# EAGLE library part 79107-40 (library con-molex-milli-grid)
RECEPTACAL
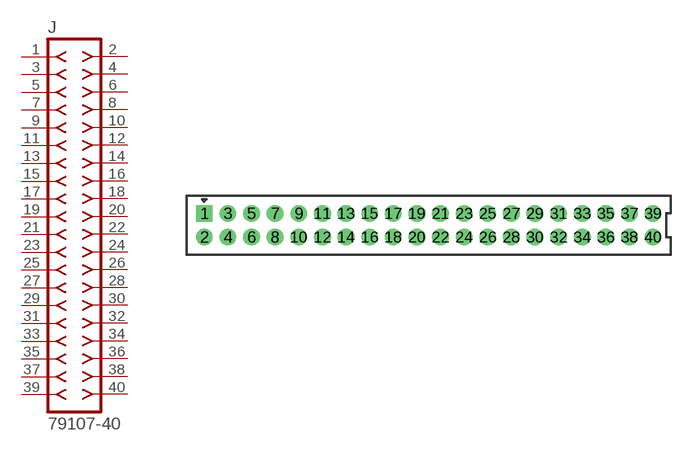
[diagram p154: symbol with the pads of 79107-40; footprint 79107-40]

Designator prefix J

## 79107-40  [79107-40]
1  1  pas
2  2  pas
3  3  pas
4  4  pas
5  5  pas
6  6  pas
7  7  pas
8  8  pas
9  9  pas
10  10  pas
11  11  pas
12  12  pas
13  13  pas
14  14  pas
15  15  pas
16  16  pas
17  17  pas
18  18  pas
19  19  pas
20  20  pas
21  21  pas
22  22  pas
23  23  pas
24  24  pas
25  25  pas
26  26  pas
27  27  pas
28  28  pas
29  29  pas
30  30  pas
31  31  pas
32  32  pas
33  33  pas
34  34  pas
35  35  pas
36  36  pas
37  37  pas
38  38  pas
39  39  pas
40  40  pas

## Footprint 79107-40 (pad centres in mm)
RECEPTACAL Dual Row, Vertical, Through-Hole
drill 0.914 square: 1 -19,1
drill 0.914: 2 -19,-1; 3 -17,1; 4 -17,-1; 5 -15,1; 6 -15,-1; 7 -13,1; 8 -13,-1; 9 -11,1; 10 -11,-1; 11 -9,1; 12 -9,-1; 13 -7,1; 14 -7,-1; 15 -5,1; 16 -5,-1; 17 -3,1; 18 -3,-1; 19 -1,1; 20 -1,-1; 21 1,1; 22 1,-1; 23 3,1; 24 3,-1; 25 5,1; 26 5,-1; 27 7,1; 28 7,-1; 29 9,1; 30 9,-1; 31 11,1; 32 11,-1; 33 13,1; 34 13,-1; 35 15,1; 36 15,-1; 37 17,1; 38 17,-1; 39 19,1; 40 19,-1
